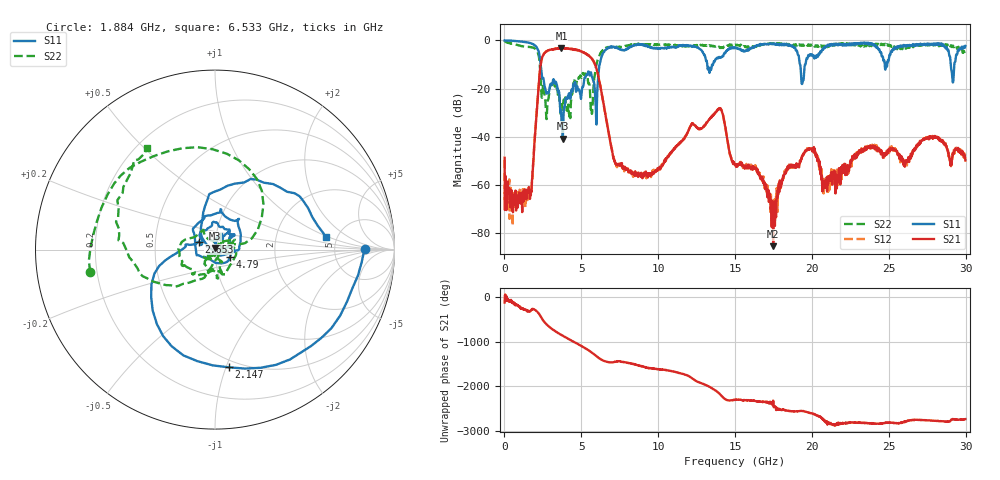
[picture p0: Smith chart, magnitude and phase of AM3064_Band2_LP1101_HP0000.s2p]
# Hz S DB R 50.0
!freq dBS11 angS11 dBS21 angS21 dBS12 angS12 dBS22 angS22
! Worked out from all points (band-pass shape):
!   1600 points, 10 MHz to 29.98 GHz, reference 50 ohm
!   highest |S21| = -3.18 dB at 3.703 GHz (marker M1); lowest = -85.5 dB at 17.48 GHz (marker M2)
!   |S21| within 3 dB of the highest: 2.518 GHz to 5.458 GHz (2.94 GHz wide, 73.7 % of centre)
!   lowest |S11| = -40.8 dB at 3.796 GHz (marker M3), VSWR 1.02, Z = 50 + j0.917 ohm
!   |S11| at or under -10 dB: 2.357 GHz to 6.189 GHz (3.832 GHz wide, 89.7 % of centre); 13.19 GHz to 13.51 GHz (315.3 MHz wide, 2.36 % of centre); 19.22 GHz to 19.58 GHz (356.6 MHz wide, 1.84 % of centre)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
!   |S22| runs from -32.7 to -0.2 dB; largest |S21 - S12| = 0.022
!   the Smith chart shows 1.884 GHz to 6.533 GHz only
!   S11 on the Smith chart (normalised r, x): 1.884 GHz: 11, +0; 2.147 GHz: 0.44, -1.02; 2.653 GHz: 0.83, +0.08; 4.79 GHz: 1.17, -0.10; 6.533 GHz: 4.08, +0.90
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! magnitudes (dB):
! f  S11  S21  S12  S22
! 10 MHz  0.0  -48.8  -49.6  -0.2
! 684.8 MHz  -0.2  -65.4  -69.2  -1.7
! 1.641 GHz  -1.0  -63.8  -64.4  -2.8
! 1.884 GHz  -1.6  -49.3  -48.8  -3.0
! 2.147 GHz  -3.6  -25.0  -24.9  -4.7
! 2.653 GHz  -19.9  -5.0  -5.0  -24.6
! 3.703 GHz  -31.7  -3.2  -3.4  -26.4
! 3.796 GHz  -40.8  -3.3  -3.2  -28.0
! 4.79 GHz  -20.6  -4.1  -4.0  -16.3
! 5.015 GHz  -21.8  -4.6  -4.6  -15.6
! 5.671 GHz  -14.7  -7.5  -7.5  -29.3
! 5.952 GHz  -29.2  -11.0  -11.1  -10.9
! 6.533 GHz  -4.1  -29.5  -29.4  -3.4
! 7.283 GHz  -3.2  -51.6  -52.0  -2.7
! 10 GHz  -3.4  -53.2  -53.1  -1.8
! 13.97 GHz  -6.9  -28.6  -28.3  -2.8
! 15 GHz  -2.9  -51.8  -51.8  -1.9
! 17.48 GHz  -1.4  -85.5  -67.7  -1.3
! 19.99 GHz  -5.8  -45.0  -45.1  -1.8
! 20.83 GHz  -3.2  -61.3  -60.4  -2.2
! 25 GHz  -7.9  -45.6  -45.5  -1.8
! 29.98 GHz  -2.3  -49.9  -48.7  -4.6
